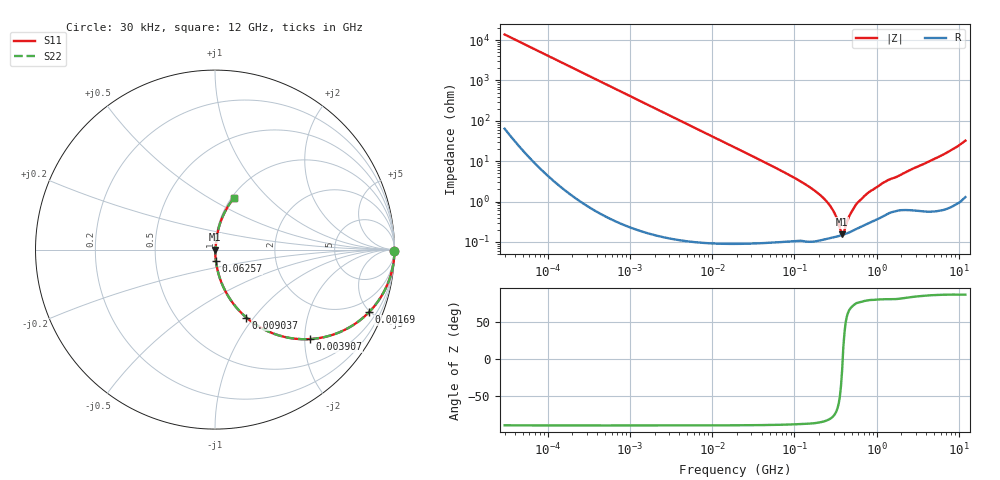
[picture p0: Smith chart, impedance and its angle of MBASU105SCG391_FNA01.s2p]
! MBASU105SCG391_FNA01  S-PARAMETER MODEL  ( General Type )
! Model Generated by TAIYO YUDEN Corporation (http://www.ty-top.com)
! Version 1.0
! TAIYO YUDEN Control No. 130207
! Copyright(c) 2013 TAIYO YUDEN CO.,LTD. All Rights Reserved.
! Product Description (link to TY-COMPAS)
! https://ds.yuden.co.jp/TYCOMPAS/or/detail?pn=MBASU105SCG391JFNA01&u=M
! Products Name : Multilayer Ceramic Capacitors
! Characteristics :
!  Capacitance : 390 pF , Rated Voltage : 50V , TCC : CG / C0G
!  Case Size : 1.0 x 0.5 / 0.039 x 0.02 [mm/inch] , Thickness : 0.5 / 0.02 [mm/inch]
!  (Conditions: Temperature = 25 degC , DC Bias Current/Voltage = 0A / 0V)
! External Node Assignments :
!  1  o---| |---o  2
! GND o---------o GND
! Frequency Range : 30000Hz  -  12GHz  [ 401 STEP ]
# MHz S RI R 50
! Freq[MHz].  S11 Real  S11 Imag  S21 Real  S21 Imag  S12 Real  S12 Imag  S22 Real  S22 Imag
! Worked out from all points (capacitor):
!   401 points, 30 kHz to 12 GHz, reference 50 ohm
!   read as one part in series: C = 384 pF near 32 kHz
!   lowest |Z| = 153 mohm at 380.7 MHz (marker M1)
!   series resonance near 386.8 MHz, so ESL is about 440 pH
!   S11 on the Smith chart (normalised r, x): 30 kHz: open; 1.69 MHz: 1.00, -4.91; 3.907 MHz: 1.00, -2.12; 9.037 MHz: 1.00, -0.92; 62.57 MHz: 1.00, -0.13; 12 GHz: 1.03, +0.65
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0.03  0.9999 -0.00723  8.57e-05 0.00723  8.57e-05 0.00723  0.9999 -0.00723
0.260295  0.996 -0.0625  0.00396 0.0625  0.00396 0.0625  0.996 -0.0625
0.831097  0.9613 -0.1926  0.0387 0.1926  0.0387 0.1926  0.9613 -0.1926
1.689526  0.8575 -0.3492  0.1425 0.3492  0.1425 0.3492  0.8575 -0.3492
2.258455  0.7711 -0.4197  0.2289 0.4197  0.2289 0.4197  0.7711 -0.4197
3.907499  0.5297 -0.4986  0.4703 0.4986  0.4703 0.4986  0.5297 -0.4986
9.037177  0.1743 -0.3784  0.8257 0.3784  0.8257 0.3784  0.1743 -0.3784
18.97367  0.0462 -0.2078  0.9538 0.2078  0.9538 0.2078  0.0462 -0.2078
62.56649  0.00511 -0.0642  0.9949 0.0642  0.9949 0.0642  0.00511 -0.0642
164.6252  0.00143 -0.0206  0.9986 0.0206  0.9986 0.0206  0.00143 -0.0206
220.0608  0.00128 -0.0127  0.9987 0.0127  0.9987 0.0127  0.00128 -0.0127
275.7901  0.0013 -0.0074  0.9987 0.0074  0.9987 0.0074  0.0013 -0.0074
313.7612  0.00134 -0.00454  0.9987 0.00454  0.9987 0.00454  0.00134 -0.00454
356.9603  0.00142 -0.00176  0.9986 0.00176  0.9986 0.00176  0.00142 -0.00176
380.7415  0.00148 -0.000392  0.9985 0.000392  0.9985 0.000392  0.00148 -0.000392
406.107  0.00155 0.0011  0.9985 -0.0011  0.9985 -0.0011  0.00155 0.0011
492.8008  0.00184 0.00513  0.9982 -0.00513  0.9982 -0.00513  0.00184 0.00513
598.0015  0.00229 0.00943  0.9977 -0.00943  0.9977 -0.00943  0.00229 0.00943
799.3715  0.00315 0.0165  0.9968 -0.0165  0.9968 -0.0165  0.00315 0.0165
1428.372  0.00635 0.0343  0.9936 -0.0343  0.9936 -0.0343  0.00635 0.0343
5534.236  0.0208 0.1214  0.9792 -0.1214  0.9792 -0.1214  0.0208 0.1214
12000  0.1037 0.2855  0.8963 -0.2855  0.8963 -0.2855  0.1037 0.2855
